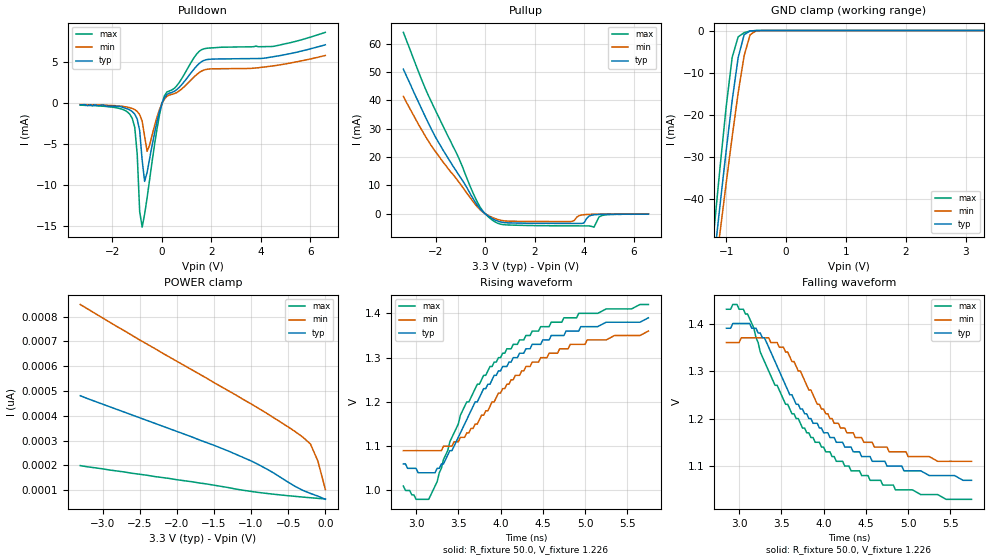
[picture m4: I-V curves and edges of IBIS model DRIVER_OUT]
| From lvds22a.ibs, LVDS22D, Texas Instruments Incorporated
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|   Driver Output  MODEL
[Model]   DRIVER_OUT
Model_type   3-state
| Signals   1Y,1Z,2Y,2Z
Vmeas = 1.2V   |Reference voltage for timing measurements
Cref = 5pF   |Timing specification test load capacitance value
Rref = 50   |Note: 50 Ohm load; single ended configuration
| variable   typ   min   max
C_comp   3.66pF   3.58pF   3.88pF
|   typ   min   max
[Temperature Range]   25.0   -40   85
[Voltage range]   3.3V   3.0V   3.6V
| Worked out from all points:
|   slope of the pulldown table from 0 to 0.495 V, typ, clamps not added: 333 ohm
|   slope of the pullup table from 0 to 0.495 V, typ, clamps not added: 192 ohm
|   GND clamp passes 1 mA (typ) near -0.70 V on its own axis
|   rising waveform, R_fixture 50.0, V_fixture 1.226: 20-80 % time 845ps typ, 880ps min, 842ps max; typ from 1.06 V to 1.39 V
|   falling waveform, R_fixture 50.0, V_fixture 1.226: 20-80 % time 930ps typ, 700ps min, 987ps max; typ from 1.39 V to 1.07 V
[Pulldown]
|   Voltage   I(typ)   I(min)   I(max)
-3.3V     -200uA     -160uA     -250uA
-1.2V     -1.03mA    -649uA     -1.86mA
-1.1V     -1.34mA    -789uA     -2.95mA
-1V       -1.95mA    -1.01mA    -6.25mA
-900mV    -3.37mA    -1.4mA     -13.3mA
-800mV    -6.98mA    -2.21mA    -15.2mA
-700mV    -9.59mA    -4.08mA    -13.6mA
-600mV    -8.48mA    -5.89mA    -11.6mA
-200mV    -2.26mA    -1.71mA    -3.15mA
100mV     665uA      504uA      905uA
1.5V      4.86mA     3.75mA     6.35mA
6.6V      7.16mA     5.85mA     8.69mA
[Pullup]
|   Voltage   I(typ)   I(min)   I(max)
| Note that the[Pullup]voltage table is referenced to Vcc
| and is calculated using Vtable=Vcc - Vmeasured.
-3.3V     51mA       41.4mA     64mA
-2.4V     34mA       27.2mA     43.9mA
-1.7V     22.5mA     18.3mA     31mA
-1.1V     14.2mA     11.7mA     20.4mA
-300mV    2.88mA     2.34mA     3.95mA
300mV     -1.72mA    -1.33mA    -2.28mA
800mV     -3.14mA    -2.52mA    -3.88mA
3.5V      -3.41mA    -2.73mA    -4.26mA
3.9V      -3.42mA    -427uA     -4.27mA
4.4V      -370uA     -164uA     -4.72mA
4.7V      -210uA     -120uA     -676uA
6.6V      -100uA     -70uA      -100uA
[GND_clamp]
|   Voltage   I(typ)   I(min)   I(max)
| Outputs in High Impedance (off)
-3.6V     -391mA     -362mA     -433mA
-1.3V     -67.3mA    -71.1mA    -62mA
-1.2V     -54.1mA    -59.3mA    -46.9mA
-1.1V     -41.1mA    -47.6mA    -32.1mA
-1V       -28.5mA    -36.2mA    -18.1mA
-900mV    -16.6mA    -25.2mA    -6.38mA
-800mV    -6.42mA    -14.8mA    -1.5mA
-700mV    -997uA     -5.97mA    -506uA
-600mV    -101uA     -992uA     -108uA
-500mV    -8.6uA     -72.8uA    -9.14uA
3.3V      62.9pA     313pA      54pA
[POWER_clamp]
|   Voltage   I(typ)   I(min)   I(max)
| Note that the [POWER_clamp] voltage table is referenced to Vcc
| and is calculated using Vtable = Vcc - Vmeasured.
| Outputs in Tri-state.
-3.3V     481pA      849pA      199pA
-2.5V     392pA      706pA      164pA
-1.3V     257pA      500pA      110pA
-900mV    203pA      430pA      90.7pA
-700mV    170pA      393pA      83.7pA
-500mV    132pA      355pA      77.5pA
-300mV    98.7pA     313pA      71.9pA
-200mV    86.7pA     286pA      69.3pA
-100mV    75.9pA     217pA      66.9pA
0V        62.9pA     103pA      64.5pA
[Ramp]
|   typ   min   max
dV/dt_r   0.201/880ps   0.162/921ps   0.250/884ps
dV/dt_f   0.200/997ps   0.160/852ps   0.249/1.056ns
R_load = 50ohm | Note: Simulation with 100 ohm load and 10pF C load.
[Rising Waveform]
R_fixture = 50.0
V_fixture = 1.226
V_fixture_min = 1.229
V_fixture_max = 1.218
C_fixture = 0p
L_fixture = 0n
|   V(typ)  V(min)  V(max)
2.85ns    1.06V      1.09V      1.01V
3ns       1.05V      1.09V      980mV
3.15ns    1.04V      1.09V      980mV
3.325ns   1.06V      1.1V       1.07V
3.6ns     1.16V      1.13V      1.2V
3.8ns     1.23V      1.17V      1.26V
4.075ns   1.28V      1.24V      1.32V
4.375ns   1.33V      1.29V      1.36V
4.825ns   1.36V      1.33V      1.39V
5.75ns    1.39V      1.36V      1.42V
[Falling Waveform]
R_fixture = 50.0
V_fixture = 1.226
V_fixture_min = 1.229
V_fixture_max = 1.218
C_fixture = 0p
L_fixture = 0n
|   V(typ)  V(min)  V(max)
2.85ns    1.39V      1.36V      1.43V
2.975ns   1.4V       1.36V      1.44V
3.1ns     1.4V       1.37V      1.42V
3.3ns     1.37V      1.37V      1.32V
3.45ns    1.31V      1.36V      1.27V
3.675ns   1.23V      1.31V      1.2V
3.925ns   1.19V      1.23V      1.15V
4.15ns    1.15V      1.19V      1.11V
4.775ns   1.1V       1.13V      1.06V
5.75ns    1.07V      1.11V      1.03V
